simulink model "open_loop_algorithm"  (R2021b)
settings: Solver=FixedStepAuto  StartTime=0.0  StopTime=10.0  RelTol=1e-3  EnableMultiTasking=on
InitFcn:
  | open_loop_data;
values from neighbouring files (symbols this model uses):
  Ts = 1 / PWM_frequency    (= 5e-05)    [open_loop_data.m]    (also in foc_qep_data.m; qep_calibration_data.m)
undefined symbols (not defined in the file or in its folder): DiscIntNeverNeededParam, motor
libraries: mcbcontrolslib x2

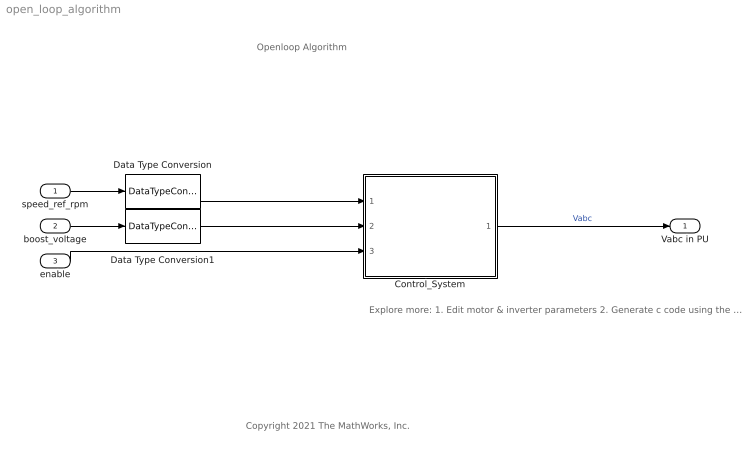
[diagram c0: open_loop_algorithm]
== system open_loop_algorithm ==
  note: Openloop Algorithm
  note: Explore more: 1. Edit motor & inverter parameters 2. Generate c code using the 'Embedded Coder' app 3. Integrate generated code with driver code 4. Control motor via host model
  note: Copyright 2021 The MathWorks, Inc.
  speed_ref_rpm : Inport  OutDataTypeStr=single  PortDimensions=1
  boost_voltage : Inport  Port=2  OutDataTypeStr=single  PortDimensions=1
  enable : Inport  Port=3  OutDataTypeStr=boolean  PortDimensions=1
  Control_System : Subsystem
  Data Type Conversion : DataTypeConversion  OutDataTypeStr=dataType
  Data Type Conversion1 : DataTypeConversion  OutDataTypeStr=dataType
  Vabc in PU : Outport
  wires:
  boost_voltage/1 -> Data Type Conversion1/1
  speed_ref_rpm/1 -> Data Type Conversion/1
  Data Type Conversion/1 -> Control_System/1(Speed_ref)
  Data Type Conversion1/1 -> Control_System/2(LowerSaturation)
  enable/1 -> Control_System/3(enable)
  Control_System/1(Vabc in PU) -> Vabc in PU/1  "Vabc"

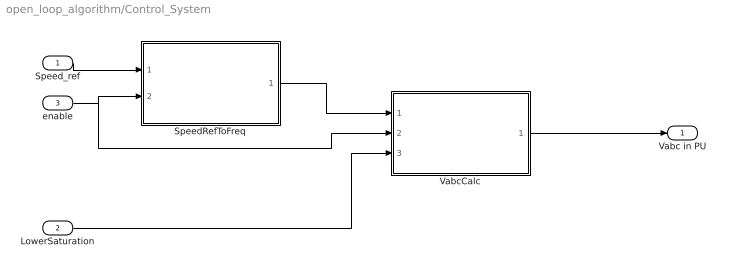
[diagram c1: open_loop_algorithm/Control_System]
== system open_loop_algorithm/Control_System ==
  Speed_ref : Inport
  LowerSaturation : Inport  Port=2
  enable : Inport  Port=3
  SpeedRefToFreq : Subsystem
  VabcCalc : Subsystem
  Vabc in PU : Outport  VectorParamsAs1DForOutWhenUnconnected=off
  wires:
  Speed_ref/1 -> SpeedRefToFreq/1(Speed_Ref)
  SpeedRefToFreq/1(Frequency) -> VabcCalc/1(Frequency)
  VabcCalc/1(Vabc) -> Vabc in PU/1
  LowerSaturation/1 -> VabcCalc/3(LowerSaturation)
  enable/1 -> VabcCalc/2(enable), SpeedRefToFreq/2(enable)

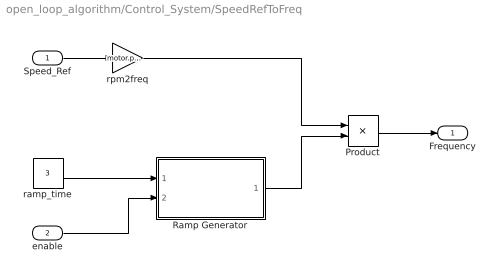
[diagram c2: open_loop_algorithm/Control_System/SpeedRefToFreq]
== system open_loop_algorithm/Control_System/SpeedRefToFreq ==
  Speed_Ref : Inport
  enable : Inport  Port=2  OutDataTypeStr=boolean
  Product : Product  RndMeth=Simplest
  Ramp Generator : Subsystem
  ramp_time : Constant  Value=3  OutDataTypeStr=dataType  SampleTime=-1
  rpm2freq : Gain  Gain=motor.polePairs/60  OutDataTypeStr=dataType  RndMeth=Simplest
  Frequency : Outport
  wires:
  Product/1 -> Frequency/1
  Ramp Generator/1(Ramp) -> Product/2
  ramp_time/1 -> Ramp Generator/1(Ramp_Time)
  enable/1 -> Ramp Generator/2(Enable)
  Speed_Ref/1 -> rpm2freq/1
  rpm2freq/1 -> Product/1

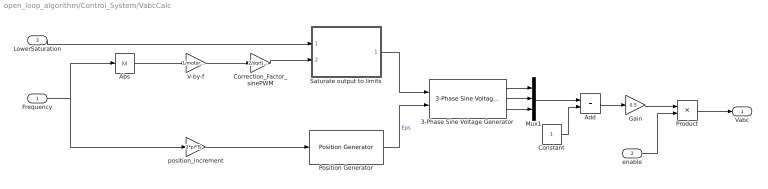
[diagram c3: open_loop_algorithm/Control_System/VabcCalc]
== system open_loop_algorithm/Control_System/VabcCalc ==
  Frequency : Inport
  enable : Inport  Port=2
  LowerSaturation : Inport  Port=3
  3-Phase Sine Voltage Generator : mcbcontrolslib/3-Phase Sine Voltage Generator  AngleInput=Per-unit  N_points=1024
  Abs : Abs  RndMeth=Simplest
  Add : Sum
  Constant : Constant  OutDataTypeStr=dataType
  Correction_Factor_sinePWM : Gain  Gain=2/sqrt(3)  RndMeth=Simplest
  Gain : Gain  Gain=0.5  RndMeth=Simplest
  Mux1 : Mux  Inputs=3
  Position Generator : mcbcontrolslib/Position Generator  AngleOutput=Per-unit  ThetaSource=External  ThetaInput=5e-4  DataType=double  ExternalReset=none
  Product : Product
  Saturate output to limits : Subsystem
  V-by-f : Gain  Gain=1/motor.base_freq  RndMeth=Simplest
  position_increment : Gain  Gain=2*pi*Ts  RndMeth=Simplest
  Vabc : Outport
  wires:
  Frequency/1 -> Abs/1, position_increment/1
  position_increment/1 -> Position Generator/1
  3-Phase Sine Voltage Generator/3 -> Mux1/3
  3-Phase Sine Voltage Generator/2 -> Mux1/2
  V-by-f/1 -> Correction_Factor_sinePWM/1
  3-Phase Sine Voltage Generator/1 -> Mux1/1
  Correction_Factor_sinePWM/1 -> Saturate output to limits/2(Vamplitude)
  LowerSaturation/1 -> Saturate output to limits/1(Lower Saturation)
  Saturate output to limits/1(Amplitude) -> 3-Phase Sine Voltage Generator/1
  Position Generator/1 -> 3-Phase Sine Voltage Generator/2  "Eps"
  Abs/1 -> V-by-f/1
  enable/1 -> Product/2
  Product/1 -> Vabc/1
  Mux1/1 -> Add/1
  Constant/1 -> Add/2
  Add/1 -> Gain/1
  Gain/1 -> Product/1

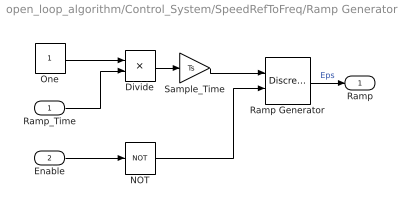
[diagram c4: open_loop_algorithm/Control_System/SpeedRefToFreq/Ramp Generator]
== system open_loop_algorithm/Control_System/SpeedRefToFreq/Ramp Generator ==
  Ramp_Time : Inport
  Enable : Inport  Port=2
  Divide : Product  Inputs=*/  RndMeth=Simplest
  NOT : Logic  Operator=NOT  IconShape=distinctive  AllPortsSameDT=off  OutDataTypeStr=boolean
  One : Constant  OutDataTypeStr=dataType  SampleTime=-1
  Ramp Generator : DiscreteIntegrator  IntegratorMethod=Accumulation: Forward Euler  gainval=1  ExternalReset=sampled level  SampleTime=-1  OutDataTypeStr=dataType  RndMeth=Simplest  LimitOutput=on  UpperSaturationLimit=1  LowerSaturationLimit=0  ICPrevOutput=DiscIntNeverNeededParam  ICPrevScaledInput=DiscIntNeverNeededParam
  Sample_Time : Gain  Gain=Ts  RndMeth=Simplest
  Ramp : Outport
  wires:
  Divide/1 -> Sample_Time/1
  Ramp Generator/1 -> Ramp/1  "Eps"
  Sample_Time/1 -> Ramp Generator/1
  One/1 -> Divide/1
  Ramp_Time/1 -> Divide/2
  Enable/1 -> NOT/1
  NOT/1 -> Ramp Generator/2

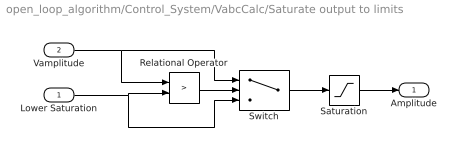
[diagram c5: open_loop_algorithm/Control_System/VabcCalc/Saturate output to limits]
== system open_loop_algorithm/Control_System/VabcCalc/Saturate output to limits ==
  Lower Saturation : Inport
  Vamplitude : Inport  Port=2
  Relational Operator : RelationalOperator  Operator=>  OutDataTypeStr=boolean  RndMeth=Simplest
  Saturation : Saturate  UpperLimit=0.95  LowerLimit=0  RndMeth=Simplest
  Switch : Switch  Criteria=u2 > Threshold
  Amplitude : Outport
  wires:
  Saturation/1 -> Amplitude/1
  Switch/1 -> Saturation/1
  Relational Operator/1 -> Switch/2
  Lower Saturation/1 -> Switch/3, Relational Operator/2
  Vamplitude/1 -> Switch/1, Relational Operator/1
